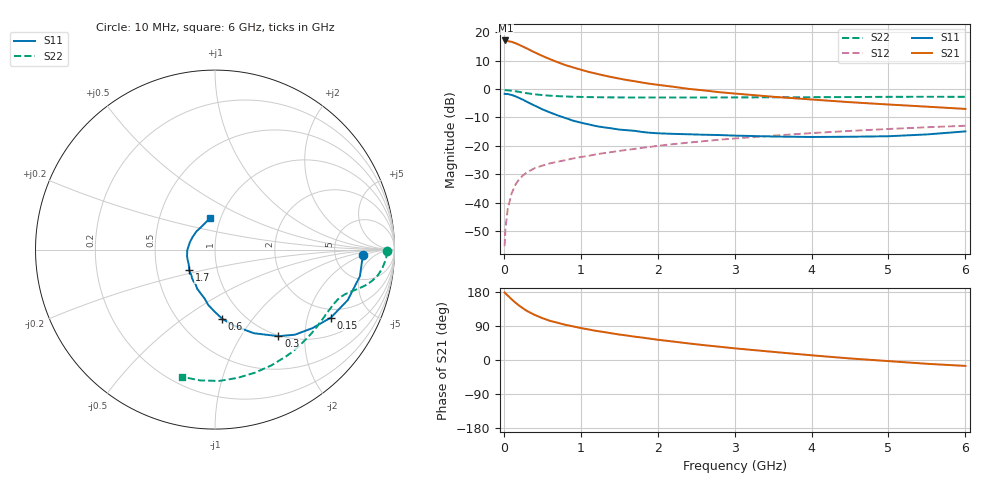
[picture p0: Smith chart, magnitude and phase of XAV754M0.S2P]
! SIEMENS Discrete & RF Semiconductors
! BFY180
! Si NPN RF Bipolar Junction Transistor in MICRO-X
! VCE = 0.75 V  IC = 4 mA
! Common Emitter S-Parameters:  May  1997
# GHz  S  MA  R  50
!  f  S11  S21  S12  S22
! GHz  MAG  ANG  MAG  ANG  MAG  ANG  MAG  ANG
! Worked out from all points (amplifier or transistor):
!   36 points, 10 MHz to 6 GHz, reference 50 ohm
!   highest |S21| = 17.2 dB at 20 MHz (marker M1)
!   |S21| within 3 dB of that: start of sweep to 313.1 MHz
!   unconditionally stable (mu >= 1): start of sweep to 11.97 MHz; 465.2 MHz to end of sweep
!   at 250 MHz: K = 0.61, MSG = 22.7 dB, |S12| = -30.4 dB
!   at 1.4 GHz: K = 1.89, MAG = 7.8 dB, |S12| = -22.2 dB
!   at 6 GHz: K = 2.14, MAG = -3.1 dB, |S12| = -12.9 dB
!   S11 on the Smith chart (normalised r, x): 10 MHz: 10, -2; 150 MHz: 1.63, -2.82; 300 MHz: 0.99, -1.48; 600 MHz: 0.79, -0.72; 1.7 GHz: 0.73, -0.17; 6 GHz: 0.89, +0.33
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0.01  0.8276 -2.2  7.115 178.2  0.0017 79.5  0.9571 -0.5
0.02  0.822 -4.3  7.224 175.9  0.0034 92.0  0.9583 -1.3
0.05  0.8208 -10.4  7.036 170.2  0.0076 80.2  0.9536 -3.3
0.1  0.7915 -20.8  6.841 160.5  0.0143 77.3  0.9378 -6.4
0.15  0.7486 -30.4  6.482 151.4  0.0206 71.5  0.9183 -9.0
0.2  0.6977 -38.8  6.045 143.4  0.0259 67.3  0.8944 -11.1
0.25  0.6504 -46.8  5.612 136.2  0.0302 62.8  0.8695 -12.9
0.3  0.5979 -53.8  5.221 129.5  0.0341 59.4  0.847 -14.2
0.4  0.5136 -65.1  4.458 119.1  0.0403 55.8  0.8121 -16.1
0.5  0.4411 -75.3  3.858 110.5  0.0447 52.5  0.7855 -17.6
0.6  0.3879 -84.0  3.377 103.3  0.0491 51.1  0.7666 -18.9
0.8  0.3099 -97.1  2.658 92.8  0.0559 50.4  0.7425 -21.4
1  0.2567 -108.2  2.206 84.4  0.0636 49.5  0.7294 -24.2
1.1  0.2394 -114.5  2.02 80.7  0.0665 49.7  0.7243 -25.6
1.4  0.2035 -129.2  1.63 70.4  0.0777 49.4  0.7156 -30.2
1.7  0.1841 -141.3  1.38 61.6  0.0883 48.4  0.7114 -35.0
2.2  0.1627 -159.5  1.103 48.7  0.1072 46.3  0.712 -43.3
2.8  0.155 -178.3  0.884 35.1  0.1282 43.0  0.714 -53.0
3.5  0.1461 163.9  0.734 21.5  0.1514 38.2  0.7173 -64.1
4.5  0.1447 135.5  0.589 4.1  0.1834 30.2  0.7257 -80.0
5.5  0.159 109.2  0.491 -10.0  0.2128 22.0  0.7335 -96.4
6  0.1799 98.2  0.448 -15.6  0.2261 17.5  0.7323 -104.5
